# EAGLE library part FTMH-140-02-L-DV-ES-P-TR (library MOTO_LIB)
MICRO SOCKET, 1.0MM, SMD, 2X40WAY, MALE
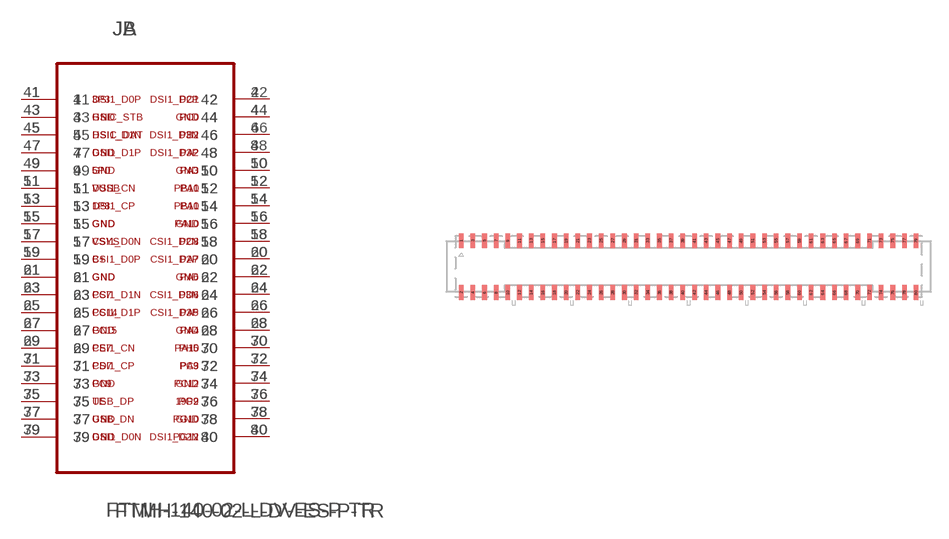
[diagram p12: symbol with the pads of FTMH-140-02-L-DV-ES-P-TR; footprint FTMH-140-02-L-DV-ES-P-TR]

Designator prefix J; gates A=FTMH-140-02-L-DV-ES-P-TR_A B=FTMH-140-02-L-DV-ES-P-TR_B

## FTMH-140-02-L-DV-ES-P-TR (MPN: ASP-193073-01; SUPPLIER: SAMTEC)  [FTMH-140-02-L-DV-ES-P-TR]
1  A:1  pas
2  A:2  pas
3  A:3  pas
4  A:4  pas
5  A:5  pas
6  A:6  pas
7  A:7  pas
8  A:8  pas
9  A:9  pas
10  A:10  pas
11  A:11  pas
12  A:12  pas
13  A:13  pas
14  A:14  pas
15  A:15  pas
16  A:16  pas
17  A:17  pas
18  A:18  pas
19  A:19  pas
20  A:20  pas
21  A:21  pas
22  A:22  pas
23  A:23  pas
24  A:24  pas
25  A:25  pas
26  A:26  pas
27  A:27  pas
28  A:28  pas
29  A:29  pas
30  A:30  pas
31  A:31  pas
32  A:32  pas
33  A:33  pas
34  A:34  pas
35  A:35  pas
36  A:36  pas
37  A:37  pas
38  A:38  pas
39  A:39  pas
40  A:40  pas
41  B:41  pas
42  B:42  pas
43  B:43  pas
44  B:44  pas
45  B:45  pas
46  B:46  pas
47  B:47  pas
48  B:48  pas
49  B:49  pas
50  B:50  pas
51  B:51  pas
52  B:52  pas
53  B:53  pas
54  B:54  pas
55  B:55  pas
56  B:56  pas
57  B:57  pas
58  B:58  pas
59  B:59  pas
60  B:60  pas
61  B:61  pas
62  B:62  pas
63  B:63  pas
64  B:64  pas
65  B:65  pas
66  B:66  pas
67  B:67  pas
68  B:68  pas
69  B:69  pas
70  B:70  pas
71  B:71  pas
72  B:72  pas
73  B:73  pas
74  B:74  pas
75  B:75  pas
76  B:76  pas
77  B:77  pas
78  B:78  pas
79  B:79  pas
80  B:80  pas

## Footprint FTMH-140-02-L-DV-ES-P-TR (pad centres in mm)
smd 0.4 x 1.263: 1 -19.5,2.223; 2 -19.5,-2.223; 3 -18.5,2.223; 4 -18.5,-2.223; 5 -17.5,2.223; 6 -17.5,-2.223; 7 -16.5,2.223; 8 -16.5,-2.223; 9 -15.5,2.223; 10 -15.5,-2.223; 11 -14.5,2.223; 12 -14.5,-2.223; 13 -13.5,2.223; 14 -13.5,-2.223; 15 -12.5,2.223; 16 -12.5,-2.223; 17 -11.5,2.223; 18 -11.5,-2.223; 19 -10.5,2.223; 20 -10.5,-2.223; 21 -9.5,2.223; 22 -9.5,-2.223; 23 -8.5,2.223; 24 -8.5,-2.223; 25 -7.5,2.223; 26 -7.5,-2.223; 27 -6.5,2.223; 28 -6.5,-2.223; 29 -5.5,2.223; 30 -5.5,-2.223; 31 -4.5,2.223; 32 -4.5,-2.223; 33 -3.5,2.223; 34 -3.5,-2.223; 35 -2.5,2.223; 36 -2.5,-2.223; 37 -1.5,2.223; 38 -1.5,-2.223; 39 -0.5,2.223; 40 -0.5,-2.223; 41 0.5,2.223; 42 0.5,-2.223; 43 1.5,2.223; 44 1.5,-2.223; 45 2.5,2.223; 46 2.5,-2.223; 47 3.5,2.223; 48 3.5,-2.223; 49 4.5,2.223; 50 4.5,-2.223; 51 5.5,2.223; 52 5.5,-2.223; 53 6.5,2.223; 54 6.5,-2.223; 55 7.5,2.223; 56 7.5,-2.223; 57 8.5,2.223; 58 8.5,-2.223; 59 9.5,2.223; 60 9.5,-2.223; 61 10.5,2.223; 62 10.5,-2.223; 63 11.5,2.223; 64 11.5,-2.223; 65 12.5,2.223; 66 12.5,-2.223; 67 13.5,2.223; 68 13.5,-2.223; 69 14.5,2.223; 70 14.5,-2.223; 71 15.5,2.223; 72 15.5,-2.223; 73 16.5,2.223; 74 16.5,-2.223; 75 17.5,2.223; 76 17.5,-2.223; 77 18.5,2.223; 78 18.5,-2.223; 79 19.5,2.223; 80 19.5,-2.223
